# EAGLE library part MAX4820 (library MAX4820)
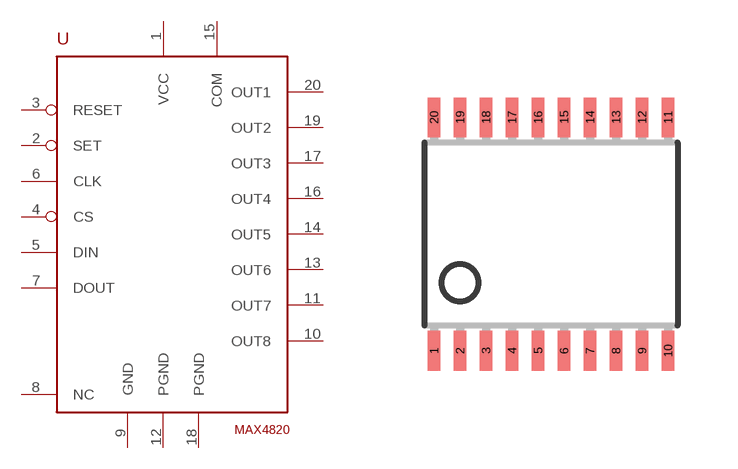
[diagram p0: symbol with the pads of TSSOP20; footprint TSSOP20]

Designator prefix -

## MAX4820  [TSSOP20]
1  VCC  pwr
2  SET  in
3  RESET  in
4  CS  in
5  DIN  in
6  CLK  in
7  DOUT  out
8  NC  nc
9  GND  pwr
10  OUT8
11  OUT7
12  PGND
13  OUT6
14  OUT5
15  COM
16  OUT4
17  OUT3
18  PGND
19  OUT2
20  OUT1

## Footprint TSSOP20 (pad centres in mm)
smd 0.305 x 0.991: 1 -2.925,-2.918; 2 -2.275,-2.918; 3 -1.625,-2.918; 4 -0.975,-2.918; 5 -0.325,-2.918; 6 0.325,-2.918; 7 0.975,-2.918; 8 1.625,-2.918; 9 2.275,-2.918; 10 2.925,-2.918; 11 2.925,2.918; 12 2.275,2.918; 13 1.625,2.918; 14 0.975,2.918; 15 0.325,2.918; 16 -0.325,2.918; 17 -0.975,2.918; 18 -1.625,2.918; 19 -2.275,2.918; 20 -2.925,2.918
